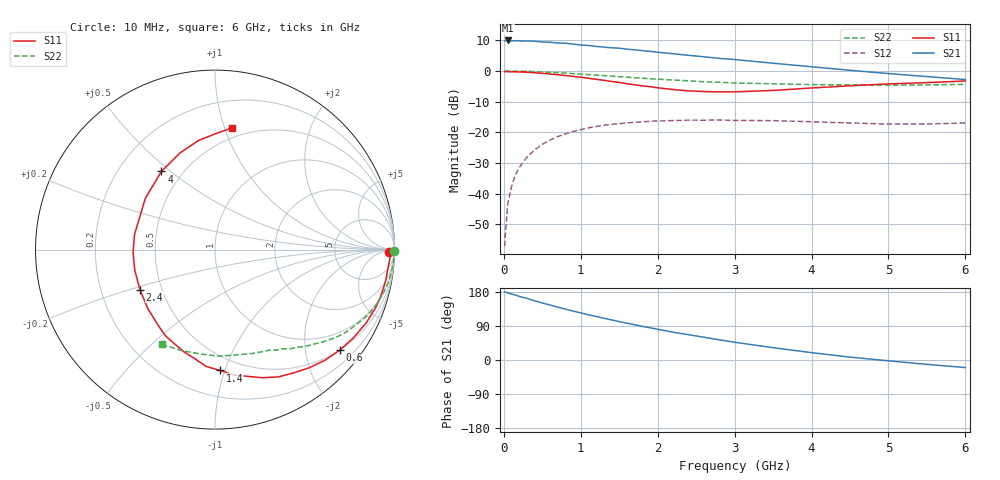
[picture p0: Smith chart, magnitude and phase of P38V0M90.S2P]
! SIEMENS Small Signal Semiconductors
! BFP181
! Si NPN RF Bipolar Junction Transistor in SOT143
! VCE = 8 V  IC = 0.9 mA
! Common Emitter S-Parameters:  March  1996
# GHz  S  MA  R  50
!  f  S11  S21  S12  S22
! GHz  MAG  ANG  MAG  ANG  MAG  ANG  MAG  ANG
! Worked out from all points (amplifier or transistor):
!   36 points, 10 MHz to 6 GHz, reference 50 ohm
!   highest |S21| = 9.9 dB at 50 MHz (marker M1)
!   |S21| within 3 dB of that: start of sweep to 1.674 GHz
!   unconditionally stable (mu >= 1): 3.371 GHz to end of sweep
!   at 250 MHz: K = 0.08, MSG = 19.7 dB, |S12| = -29.7 dB
!   at 1.4 GHz: K = 0.47, MSG = 12.5 dB, |S12| = -17.4 dB
!   at 6 GHz: K = 1.29, MAG = 3.9 dB, |S12| = -17.0 dB
!   S11 on the Smith chart (normalised r, x): 10 MHz: 59, -25; 600 MHz: 0.50, -2.75; 1.4 GHz: 0.39, -0.96; 2.4 GHz: 0.38, -0.22; 4 GHz: 0.38, +0.46; 6 GHz: 0.41, +1.06
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0.01  0.9717 -0.7  3.095 179.6  0.0014 83.2  0.9989 -0.3
0.05  0.9755 -3.0  3.139 177.1  0.0068 87.1  0.9965 -1.6
0.1  0.9687 -6.7  3.069 174.2  0.0131 83.4  0.9978 -3.2
0.15  0.9668 -10.1  3.114 171.2  0.0203 83.4  0.9943 -4.7
0.2  0.9624 -13.2  3.09 168.1  0.0266 81.6  0.9922 -6.2
0.25  0.9588 -16.4  3.059 165.2  0.0328 79.4  0.9886 -7.9
0.3  0.9522 -19.8  3.088 162.8  0.0395 76.8  0.9859 -9.3
0.4  0.9362 -25.9  3.053 156.2  0.0519 72.7  0.9772 -12.4
0.6  0.8923 -38.9  2.94 145.1  0.0751 63.7  0.9527 -18.2
0.8  0.8416 -51.5  2.828 134.3  0.0945 56.1  0.9224 -23.6
1.1  0.7606 -69.8  2.6 119.3  0.1183 45.4  0.8723 -30.7
1.4  0.6737 -87.7  2.385 105.8  0.1348 36.1  0.8228 -37.0
1.5  0.6515 -94.6  2.35 101.4  0.1388 33.7  0.8061 -38.7
1.8  0.5714 -113.3  2.142 88.8  0.1486 26.6  0.7606 -43.8
2.2  0.4984 -138.7  1.907 73.4  0.1555 18.1  0.7105 -50.1
2.4  0.4737 -152.0  1.797 66.8  0.158 14.5  0.6912 -53.2
3  0.4564 169.6  1.534 46.9  0.1566 5.9  0.6365 -61.8
3.5  0.4818 143.7  1.336 32.5  0.1551 0.9  0.6176 -69.2
4  0.5281 124.4  1.171 19.4  0.1486 -2.5  0.5992 -78.1
4.5  0.5735 109.7  1.025 7.6  0.1422 -5.1  0.5942 -87.9
5.5  0.646 89.6  0.81 -11.5  0.1372 -2.2  0.5927 -108.5
6  0.6859 81.9  0.724 -20.0  0.1419 -1.3  0.6053 -119.3
